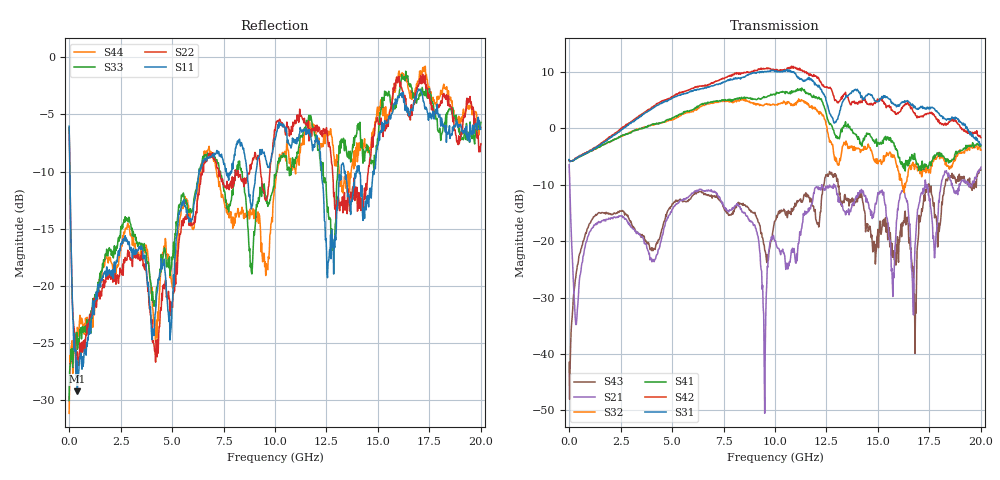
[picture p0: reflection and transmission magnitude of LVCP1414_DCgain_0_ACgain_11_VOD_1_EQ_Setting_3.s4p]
!Agilent Technologies,N5230A,MY46400459,A.07.50.48
!Agilent N5230A: A.07.50.48
!Date: Tuesday, April 17, 2012 18:30:35
!Correction: S11(Full 4 Port(1,2,3,4))
!S12(Full 4 Port(1,2,3,4))
!S13(Full 4 Port(1,2,3,4))
!S14(Full 4 Port(1,2,3,4))
!S21(Full 4 Port(1,2,3,4))
!S22(Full 4 Port(1,2,3,4))
!S23(Full 4 Port(1,2,3,4))
!S24(Full 4 Port(1,2,3,4))
!S31(Full 4 Port(1,2,3,4))
!S32(Full 4 Port(1,2,3,4))
!S33(Full 4 Port(1,2,3,4))
!S34(Full 4 Port(1,2,3,4))
!S41(Full 4 Port(1,2,3,4))
!S42(Full 4 Port(1,2,3,4))
!S43(Full 4 Port(1,2,3,4))
!S44(Full 4 Port(1,2,3,4))
!S4P File: Measurements: <S11,S12,S13,S14>,
!<S21,S22,S23,S24>,
!<S31,S32,S33,S34>,
!<S41,S42,S43,S44>:
# Hz S  dB  R 50
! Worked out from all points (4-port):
!   801 points, 300 kHz to 20 GHz, reference 50 ohm
!   strongest paths, dB at 300 kHz, 5 GHz, 10 GHz, 15 GHz, 20 GHz:
!     S31: -5.5, 5.3, 10.0, 4.7, -2.9
!     S42: -5.7, 5.6, 10.3, 5.1, -1.7
!     S41: -5.6, 1.8, 5.9, -2.5, -3.1
!     S32: -5.7, 1.5, 4.1, -6.3, -3.9
!     S21: -6.5, -14.4, -20.0, -11.4, -6.9
!     S43: -41.5, -13.4, -16.5, -17.9, -7.4
!   lowest |S11| = -29.2 dB at 400.3 MHz (marker M1), VSWR 1.07, Z = 53.3 + j1.43 ohm
!   |S11| at or under -10 dB: 37.61 MHz to 6.317 GHz (6.279 GHz wide, 198 % of centre); 12.26 GHz to 13.21 GHz (950.1 MHz wide, 7.46 % of centre); 14.09 GHz to 14.77 GHz (677.5 MHz wide, 4.69 % of centre)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
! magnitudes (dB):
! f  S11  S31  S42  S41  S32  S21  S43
! 300 kHz  -6.0  -5.5  -5.7  -5.6  -5.7  -6.5  -41.5
! 400.3 MHz  -29.2  -5.2  -5.2  -5.3  -5.2  -32.1  -24.3
! 10 GHz  -7.2  10.0  10.3  5.9  4.1  -20.0  -16.5
! 12.7 GHz  -15.5  2.4  7.1  0.8  -2.5  -10.4  -8.1
! 16.78 GHz  -3.8  3.9  2.6  -4.5  -7.3  -24.3  -29.4
! 18.05 GHz  -6.0  2.1  0.8  -5.0  -4.9  -10.5  -16.2
! 20 GHz  -6.3  -2.9  -1.7  -3.1  -3.9  -6.9  -7.4
